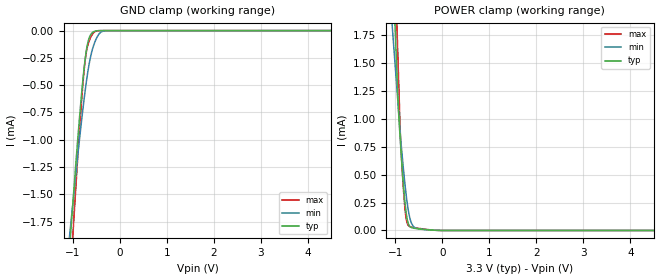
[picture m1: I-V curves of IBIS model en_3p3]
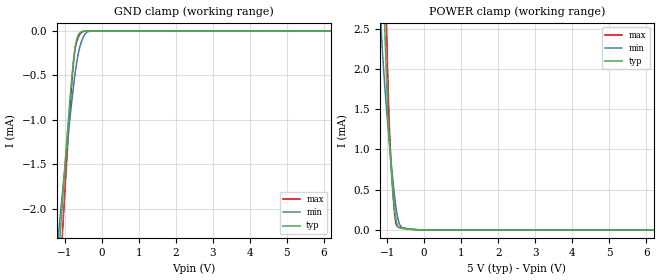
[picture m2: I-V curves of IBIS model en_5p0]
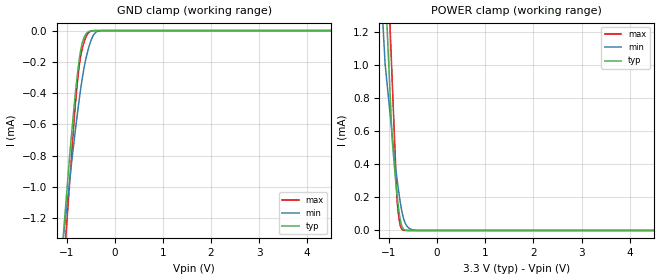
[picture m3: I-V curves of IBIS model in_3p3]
|Texas Instruments Incorporated
| ISO734x Robust EMC, Low Power, Quad-Channel Digital Isolators
| Marketing part#   Digital Voltage Range   Package-type   #pins
| ISO7340FCDW   3.0V - 5.5V   SOIC   16
[IBIS Ver]   4.1
[File name]   iso7340fc.ibs
[File Rev]   1.0
[Date]   9/29/2014
[Source]
| Texas Instruments Incorporated.
| Analog-eLab Design Center, HPA
| 12500 TI Blvd
| Dallas, TX -75243
[Notes]   Revision History:
| Rev 1.0: 9/29/2014
| - Initial version of the model.
| - Model generated from simulations in SPECTRE
| - Model matched to SPICE simulation
| - C_comp although listed in numerical order of value are
|   obtained from varying PVT conditions. For PVT conditions for
|   each specific value refer the buffer description under
|   respective [Model]. IBIS model user is responsible for using
|   appropriate C_comp to simulate for Signal Integrity.
| - Model names with a trailing _3p3 contains the model for
|   3.3V [3.0V and 3.6V]. Model names with a trailing _5p0 contains
|   the model for 5V [4.5V and 5.5V].
| - GND Clamp non monotonic for EN and IN input buffers.
| - IBIS model created from existing model of ISO7342.
[Disclaimer]
| This model is designed as an aid for customers of Texas Instruments.
| TI and its licensors and suppliers make no warranties, either expressed
| or implied, with respect to this  model, including the warranties of
| merchantability or fitness for a particular purpose. The model is
| provided solely on an "as is" basis. The entire risk as to its quality
| and performance is with the customer.
[Copyright]
(C) Copyright 2014 Texas Instruments Incorporated.All rights reserved.
|   ISO7340FCDW
[Component]   ISO7340FCDW
[Manufacturer]   TI
[Package]   |16 SOIC  -  DW package
|   typ   min   max
R_pkg   0.1228   0.0822   0.1793
L_pkg   2.2157nH   1.9245nH   2.8571nH
C_pkg   0.4645pF   0.2145pF   0.7510pF
[Pin]   signal_name   model_name   R_pin   L_pin   C_pin
1   VCC1   POWER   0.09703  2.25823nH  0.63889pF
2   GND1   GND   0.10567  2.15194nH  0.30706pF
3   INA   IN   0.12889  1.99554nH  0.21450pF
4   INB   IN   0.12623  1.94755nH  0.61276pF
5   INC   IN   0.12494  1.92646nH  0.36666pF
6   IND   IN   0.14038  2.18765nH  0.43235pF
7   NC   NC   0.17807  2.83638nH  0.45904pF
8   GND1   GND   0.08216  2.43955nH  0.44498pF
9   GND2   GND   0.10126  2.44074nH  0.40934pF
10   EN   EN   0.17928  2.85707nH  0.52717pF
11   OUTD   OUT   0.12883  1.99615nH  0.50841pF
12   OUTC   OUT   0.12617  1.94399nH  0.32633pF
13   OUTB   OUT   0.12498  1.92454nH  0.37783pF
14   OUTA   OUT   0.14050  2.18615nH  0.38097pF
15   GND2   GND   0.08275  2.09014nH  0.75096pF
16   VCC2   POWER   0.09747  2.26909nH  0.67439pF
|   Model Selectors
[Model Selector] EN
en_3p3   3.3V digital Input
en_5p0   5.0V digital Input
[Model Selector] IN
in_3p3   3.3V digital Input
in_5p0   5.0V digital Input
[Model Selector] OUT
out_3p3   3.3V digital Output
out_5p0   5.0V digital Output
| Models and submodels in the file (6): en_3p3 (Input), en_5p0 (Input), in_3p3 (Input), in_5p0 (Input), out_3p3 (3-state), out_5p0 (3-state)
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|   en_3p3 Model
[Model]   en_3p3
Model_type   Input
Vinl = 0.8
Vinh = 2
|   typ   min   max
|   (nom PVT)   (slow PVT)   (fast PVT)
C_comp   0.161pF   0.098pF   0.252pF
| Where   nom PVT is  Nominal Process, 3.3V, 27C
|   Fast PVT is Strong Process, 3.6V, -40C
|   Slow PVT is Weak Process, 3.0V, 150C
[Voltage Range]   3.3   3   3.6
[Temperature Range]   27   150   -40
[Power Clamp Reference]   3.3   3   3.6
[GND Clamp Reference]   0   0   0
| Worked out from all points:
|   GND clamp passes 1 mA (typ) near -0.90 V on its own axis
|   POWER clamp passes 1 mA (typ) near -0.92 V on its own axis
[GND Clamp]
|   Voltage   I(typ)   I(min)   I(max)
-3.3V     -16.02mA   -12.12mA   -20.07mA
-1.082V   -2.058mA   -1.927mA   -2.435mA
-933.9mV  -1.195mA   -1.301mA   -1.409mA
-815.1mV  -576.9uA   -823.1uA   -642.6uA
-775.5mV  -399.7uA   -677.1uA   -429.5uA
-735.9mV  -249.5uA   -540.6uA   -261.7uA
-696.3mV  -138.4uA   -417.2uA   -157.1uA
-656.7mV  -70.87uA   -311.6uA   -97.71uA
-547.8mV  -8.269uA   -122.2uA   -15.56uA
-438.9mV  -609.9nA   -28.59uA   -715.7nA
-300.3mV  -135.4nA   -1.693uA   -73.15nA
6.6V      0A         0A         0A
[POWER Clamp]
|   Voltage   I(typ)   I(min)   I(max)
-3.3V     37.87mA    27.97mA    46.61mA
-1.082V   2.59mA     1.912mA    3.362mA
-933.9mV  1.066mA    1.077mA    1.378mA
-894.3mV  792.6uA    854.2uA    848.9uA
-844.8mV  490.1uA    618.8uA    468.6uA
-795.3mV  245.9uA    408.6uA    190uA
-765.6mV  141.6uA    299.7uA    94.29uA
-735.9mV  76.12uA    208uA      52.02uA
-656.7mV  25.39uA    64.33uA    30.38uA
-518.1mV  15.3uA     15.27uA    20.19uA
-3.3mV    22.97nA    56.83nA    14.08nA
6.6V      0A         0A         0A
|   en_5p0 Model
[Model]   en_5p0
Model_type   Input
Vinl = 0.8
Vinh = 2
|   typ   min   max
|   (nom PVT)   (slow PVT)   (fast PVT)
C_comp   0.173pF   0.101pF   0.247pF
| Where   nom PVT is  Nominal Process, 5.0V, 27C
|   Fast PVT is Strong Process, 5.5V, -40C
|   Slow PVT is Weak Process, 4.5V, 150C
[Voltage Range]   5   4.5   5.5
[Temperature Range]   27   150   -40
[Power Clamp Reference]   5   4.5   5.5
[GND Clamp Reference]   0   0   0
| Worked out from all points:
|   GND clamp passes 1 mA (typ) near -0.90 V on its own axis
|   POWER clamp passes 1 mA (typ) near -0.92 V on its own axis
[GND Clamp]
|   Voltage   I(typ)   I(min)   I(max)
-5V       -26.85mA   -20.05mA   -33.83mA
-1.235V   -2.983mA   -2.6mA     -3.546mA
-1.13V    -2.354mA   -2.134mA   -2.795mA
-1.115V   -2.264mA   -2.068mA   -2.688mA
-1.055V   -1.904mA   -1.808mA   -2.259mA
-860mV    -799.2uA   -997uA     -914.7uA
-755mV    -317.8uA   -605uA     -335.4uA
-665mV    -81.82uA   -332uA     -109.5uA
-530mV    -5.449uA   -101.8uA   -10.68uA
-425mV    -437.8nA   -22.05uA   -447nA
-275mV    -117.8nA   -1.166uA   -60.6nA
10V       0A         0A         0A
[POWER Clamp]
|   Voltage   I(typ)   I(min)   I(max)
-5V       66.01mA    49.38mA    80.54mA
-1.235V   4.734mA    3.205mA    6.08mA
-1.13V    3.373mA    2.244mA    4.359mA
-1.085V   2.789mA    1.93mA     3.621mA
-1.055V   2.4mA      1.739mA    3.129mA
-1.025V   2.011mA    1.559mA    2.638mA
-980mV    1.427mA    1.304mA    1.9mA
-935mV    1.075mA    1.063mA    1.241mA
-845mV    491.9uA    621.1uA    470.4uA
-770mV    155.2uA    316.2uA    105.1uA
-650mV    24.69uA    59.36uA    30.24uA
10V       0A         0A         0A
|   in_3p3 Model
[Model]   in_3p3
Model_type   Input
Vinl = 0.8
Vinh = 2
|   typ   min   max
|   (nom PVT)   (slow PVT)   (fast PVT)
C_comp   0.351pF   0.323pF   0.382pF
| Where   nom PVT is  Nominal Process, 3.3V, 27C
|   Fast PVT is Strong Process, 3.6V, -40C
|   Slow PVT is Weak Process, 3.0V, 150C
[Voltage Range]   3.3   3   3.6
[Temperature Range]   27   150   -40
[Power Clamp Reference]   3.3   3   3.6
[GND Clamp Reference]   0   0   0
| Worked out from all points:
|   GND clamp passes 1 mA (typ) near -0.99 V on its own axis
|   POWER clamp passes 1 mA (typ) near -1.00 V on its own axis
[GND Clamp]
|   Voltage   I(typ)   I(min)   I(max)
-3.3V     -10.39mA   -8.115mA   -12.82mA
-1.082V   -1.37mA    -1.374mA   -1.609mA
-937.1mV  -808.8uA   -965.1uA   -983.7uA
-835.3mV  -462.9uA   -687.4uA   -545.7uA
-745.8mV  -209.8uA   -463.5uA   -250.2uA
-706.2mV  -128.4uA   -374.2uA   -164.5uA
-656.7mV  -62.3uA    -275.4uA   -96.19uA
-587.4mV  -18.62uA   -166.6uA   -35.33uA
-528mV    -5.031uA   -97.34uA   -9.656uA
-419.1mV  -267.9nA   -19.35uA   -326.7nA
-260.7mV  0A         -360nA     0A
6.6V      0A         0A         0A
[POWER Clamp]
|   Voltage   I(typ)   I(min)   I(max)
-3.3V     19.35mA    14.32mA    23.8mA
-1.241V   2.528mA    1.867mA    3.158mA
-1.082V   1.504mA    1.013mA    1.997mA
-937.1mV  563.9uA    587uA      931.8uA
-834.9mV  220.4uA    314.7uA    184.6uA
-805.2mV  142.2uA    248.2uA    99.44uA
-775.5mV  79.87uA    187.9uA    41.48uA
-745.8mV  37.68uA    135.7uA    13.04uA
-706.2mV  10.74uA    81.62uA    2.196uA
-607.2mV  291.7nA    19.75uA    21.42nA
-419.1mV  0A         452.1nA    0A
6.6V      0A         0A         0A
